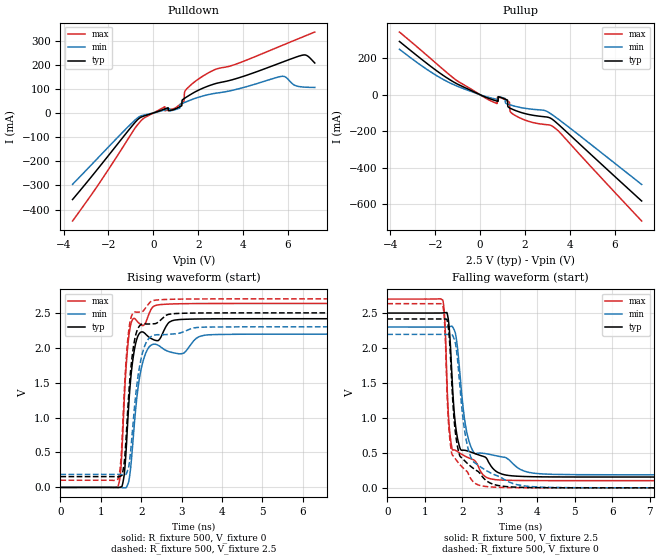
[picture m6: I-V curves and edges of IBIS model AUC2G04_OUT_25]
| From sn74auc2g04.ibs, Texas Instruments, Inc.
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[Model]   AUC2G04_OUT_25
Model_type  Output
Vref =   0
Rref =   500
Cref =   30p
Vmeas =   1.25
| variable   typ   min   max
C_comp   7.46pF   0.27pF   23.63pF
| C_pullup   8.37pF   0.27pF   23.63pF
| C_pulldown   6.54pF   1.88pF   15.77pF
[Temperature Range]   40   100   -40
| Ambient temperature   25   85   -40
[Voltage range]   2.5   2.3   2.7
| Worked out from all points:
|   slope of the pulldown table from 0 to 0.375 V, typ, clamps not added: 30.9 ohm
|   slope of the pullup table from 0 to 0.375 V, typ, clamps not added: 19.2 ohm
|   rising waveform, R_fixture 500, V_fixture 0: 20-80 % time 199ps typ, 259ps min, 159ps max; typ from 0 V to 2.42 V
|   falling waveform, R_fixture 500, V_fixture 2.5: 20-80 % time 225ps typ, 319ps min, 155ps max; typ from 2.5 V to 0.154 V
|   rising waveform, R_fixture 500, V_fixture 2.5: 20-80 % time 197ps typ, 258ps min, 157ps max; typ from 0.154 V to 2.5 V
|   falling waveform, R_fixture 500, V_fixture 0: 20-80 % time 239ps typ, 342ps min, 158ps max; typ from 2.42 V to 0 V
[Pulldown]
| AUC2G04_OUT_25
|   Voltage   I(typ)   I(min)   I(max)
-3.6V     -358.1mA   -295.3mA   -447.1mA
-445mV    -13.39mA   -9.086mA   -23.04mA
515mV     17.02mA    12.57mA    25.99mA
1.03V     19.08mA    15.52mA    23.89mA
1.27V     30.04mA    38.39mA    41.38mA
1.37V     59.36mA    42.45mA    48.97mA
1.395V    60.88mA    43.46mA    85.17mA
1.48V     65.99mA    46.82mA    98.83mA
2.545V    114.9mA    77.95mA    170.8mA
5.695V    208.5mA    151.5mA    277.9mA
6.74V     240.5mA    107.2mA    317.8mA
7.2V      207mA      105.9mA    335.2mA
[Pullup]
| AUC2G04_OUT_25
|   Voltage   I(typ)   I(min)   I(max)
-3.6V     292.7mA    249.8mA    344.4mA
-960mV    55.5mA     44.14mA    71.52mA
730mV     -33.82mA   -24.42mA   -47.21mA
760mV     -34.84mA   -25.13mA   -47.16mA
770mV     -35.18mA   -25.36mA   -13.07mA
1.115V    -23.84mA   -20.26mA   -27.67mA
1.215V    -28.81mA   -50.48mA   -34.67mA
1.295V    -71.05mA   -53.78mA   -40.2mA
1.345V    -74.3mA    -55.73mA   -93.3mA
1.755V    -94.43mA   -68.81mA   -126mA
3.305V    -143.1mA   -117.6mA   -180mA
7.2V      -583mA     -492.1mA   -692.8mA
[Ramp]
| AUC2G04_OUT_25
| variable   typ   min   max
dV/dt_r   1.45/2.00E-10   1.32/2.61E-10   1.58/1.61E-10
dV/dt_f   1.41/2.26E-10   1.28/3.25E-10   1.56/1.55E-10
R_load = 500
[Rising Waveform]
| AUC2G04_OUT_25
R_fixture =   500
C_fixture =   0
L_fixture =   0
V_fixture =   0
V_fixture_min = 0
V_fixture_max = 0
|   Time   V(typ)   V(min)   V(max)
0s        9.76nV     28.57nV    1.856nV
1.425ns   -3.642mV   492.4uV    13.7mV
1.5ns     7.583mV    -2.216mV   293.2mV
1.58ns    180.8mV    -5.41mV    1.245V
1.735ns   1.52V      258.7mV    2.316V
1.995ns   2.224V     1.683V     2.331V
2.39ns    2.102V     2.044V     2.611V
3.145ns   2.409V     1.978V     2.631V
3.91ns    2.414V     2.19V      2.634V
22ns      2.416V     2.195V     2.634V
[Falling Waveform]
| AUC2G04_OUT_25
R_fixture =   500
C_fixture =   0
L_fixture =   0
V_fixture =   2.5
V_fixture_min = 2.3
V_fixture_max = 2.7
|   Time   V(typ)   V(min)   V(max)
0s        2.5V       2.3V       2.7V
1.48ns    2.502V     2.3V       2.686V
1.54ns    2.505V     2.3V       2.331V
1.63ns    2.399V     2.302V     1.042V
1.73ns    1.549V     2.308V     556.2mV
1.89ns    666mV      1.914V     512.4mV
2.185ns   519.5mV    656.9mV    425.5mV
2.77ns    308.9mV    473.9mV    127mV
4.405ns   156.2mV    193.4mV    103.1mV
22ns      154.5mV    186.3mV    102.6mV
[Rising Waveform]
| AUC2G04_OUT_25
R_fixture =   500
C_fixture =   0
L_fixture =   0
V_fixture =   2.5
V_fixture_min = 2.3
V_fixture_max = 2.7
|   Time   V(typ)   V(min)   V(max)
0s        154.5mV    186.3mV    102.6mV
1.425ns   151.4mV    186.6mV    117.9mV
1.5ns     165.3mV    184.3mV    415.8mV
1.58ns    354.6mV    184mV      1.356V
1.65ns    942.1mV    219.3mV    2.002V
1.725ns   1.587V     443.8mV    2.374V
1.84ns    2.119V     1.181V     2.513V
1.98ns    2.325V     1.794V     2.512V
2.315ns   2.343V     2.179V     2.678V
22ns      2.5V       2.3V       2.7V
[Falling Waveform]
| AUC2G04_OUT_25
R_fixture =   500
C_fixture =   0
L_fixture =   0
V_fixture =   0
V_fixture_min = 0
V_fixture_max = 0
|   Time   V(typ)   V(min)   V(max)
0s        2.416V     2.195V     2.634V
1.48ns    2.415V     2.195V     2.612V
1.535ns   2.415V     2.195V     2.288V
1.62ns    2.329V     2.194V     1.048V
1.715ns   1.556V     2.198V     504.5mV
1.925ns   472.1mV    1.523V     340.2mV
2.155ns   340.2mV    562.5mV    210.4mV
2.495ns   190.2mV    297mV      30.95mV
4.235ns   1.877mV    7.916mV    500.7uV
22ns      20.77uV    1.816uV    9.619uV
